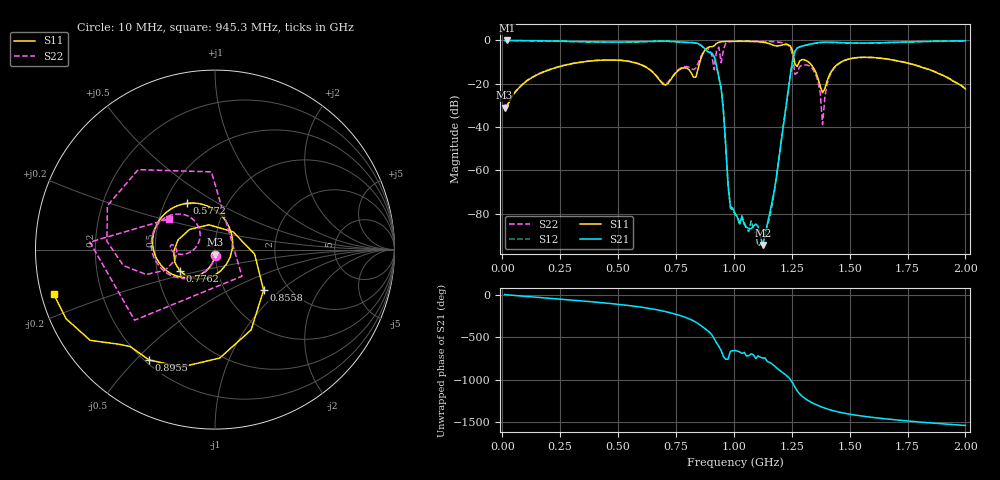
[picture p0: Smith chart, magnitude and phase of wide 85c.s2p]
!Agilent Technologies,E8363B,SG43030131,A.07.50.48
!Agilent E8363B: A.07.50.48
!Date: Monday, December 01, 2025 21:21:41
!Correction: S11(Full 2 Port(1,2))
!S21(Full 2 Port(1,2))
!S12(Full 2 Port(1,2))
!S22(Full 2 Port(1,2))
!S2P File: Measurements: S11, S21, S12, S22:
# Hz S  dB  R 50
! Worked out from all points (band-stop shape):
!   201 points, 10 MHz to 2 GHz, reference 50 ohm
!   highest |S21| = 0.01 dB at 19.95 MHz (marker M1); lowest = -94.4 dB at 1.124 GHz (marker M2)
!   |S21| within 3 dB of the highest: start of sweep to 866.9 MHz; 1.283 GHz to end of sweep
!   lowest |S11| = -31.1 dB at 10 MHz (marker M3), VSWR 1.06, Z = 50.1 - j2.8 ohm
!   |S11| at or under -10 dB: start of sweep to 342.6 MHz; 561.8 MHz to 853.4 MHz (291.5 MHz wide, 41.2 % of centre); 1.733 GHz to end of sweep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
!   |S22| runs from -38.8 to -0.3 dB; largest |S21 - S12| = 0.032
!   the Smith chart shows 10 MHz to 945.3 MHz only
!   S11 on the Smith chart (normalised r, x): 10 MHz: 1.00, -0.06; 577.1 MHz: 0.65, +0.37; 776.1 MHz: 0.66, -0.16; 855.8 MHz: 1.50, -0.78; 895.5 MHz: 0.22, -0.55; 945.3 MHz: 0.04, -0.14
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1e7  -31.07 -86.4  -0.01 -0.3  -0.05 -2.2  -29.52 -83.5
1.995e7  -30.26 -87.8  0.01 -3.1  -0.06 -4.7  -29.92 -90.6
3.483e8  -9.91 -166.7  -0.55 -76.2  -0.64 -76.3  -9.81 -163.4
5.7715e8  -10.42 121.3  -0.60 -139.7  -0.68 -139.8  -10.32 140.2
6.7665e8  -17.95 43.3  -0.32 175.8  -0.40 175.7  -17.66 130.0
7.7615e8  -12.78 -148.9  -0.75 105.8  -0.83 105.7  -12.40 -178.3
8.5575e8  -9.05 -39.9  -2.00 -1.2  -2.09 -1.3  -7.79 -160.2
8.9555e8  -2.90 -120.8  -5.61 -84.3  -5.68 -84.6  -4.18 133.9
9.254e8  -1.31 -144.0  -11.78 150.7  -11.86 150.4  -4.49 -138.7
9.453e8  -0.61 -164.5  -22.13 59.6  -22.21 59.2  -10.27 146.0
9.851e8  -0.39 166.3  -76.72 52.8  -77.52 53.1  -0.52 158.4
1.005e9  -0.38 154.1  -79.63 63.3  -80.37 53.6  -0.40 143.0
1.1244e9  -0.82 63.7  -94.38 -27.4  -92.74 -28.5  -0.38 78.2
1.1841e9  -2.53 -79.5  -62.72 -141.0  -63.01 -141.6  -0.66 35.5
1.21395e9  -1.97 -171.7  -39.05 156.7  -39.10 156.4  -1.14 0.8
1.2637e9  -10.82 82.3  -5.02 -8.2  -5.11 -8.3  -15.62 -121.1
1.29355e9  -8.84 110.9  -2.65 -111.9  -2.72 -112.0  -11.50 -154.6
1.3433e9  -12.49 74.1  -1.36 161.3  -1.44 161.1  -13.61 76.8
1.3831e9  -24.16 110.0  -0.82 114.8  -0.90 114.6  -38.79 -35.9
1.4428e9  -11.47 151.4  -0.92 65.8  -0.99 65.6  -11.77 151.2
1.67165e9  -8.74 76.8  -0.90 -25.1  -0.97 -25.4  -8.69 51.5
2e9  -22.36 39.4  -0.20 -98.3  -0.27 -98.5  -22.15 -55.7
